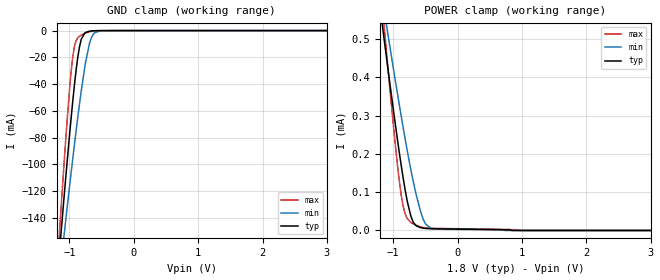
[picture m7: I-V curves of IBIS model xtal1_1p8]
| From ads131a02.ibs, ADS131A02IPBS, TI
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|   xtal1_1p8 Model
[Model]   xtal1_1p8
Model_type   Input
Vinl = 0.36
Vinh = 1.44
|   typ   min   max
|   (nom PVT)   (fast PVT)   (slow PVT)
C_comp   1.078e-12   1.074e-12   1.087e-12
| Where nom  PVT is Nominal Process, 1.8V, 27C
|   Fast PVT is Strong Process,  2V, -40C
|   Slow PVT is Weak Process,   1.65V, 125C
[Voltage Range]   1.8   1.65   2
|Junction Temperature
[Temperature Range]   27   125   -40
[Power Clamp Reference]   1.8   1.65   2
[GND Clamp Reference]   0   0   0
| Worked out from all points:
|   GND clamp passes 1 mA (typ) near -0.72 V on its own axis
[GND Clamp]
|   Voltage   I(typ)   I(min)   I(max)
-1.8V     -557.8mA   -477.6mA   -662.7mA
-1.148V   -161.8mA   -181.3mA   -146.5mA
-1.106V   -137.7mA   -162.9mA   -115.8mA
-1.055V   -108.9mA   -140.8mA   -79.9mA
-994mV    -76.12mA   -115mA     -41.72mA
-952.2mV  -54.96mA   -97.69mA   -21.36mA
-902mV    -32.17mA   -77.48mA   -8.397mA
-844.2mV  -12.42mA   -55.34mA   -4.36mA
-750.6mV  -1.441mA   -24.19mA   -1.867mA
-651.6mV  -231.6uA   -4.566mA   -469.7uA
-521.2mV  -19.95uA   -158.6uA   -32.31uA
3.6V      0A         0A         0A
[POWER Clamp]
|   Voltage   I(typ)   I(min)   I(max)
-1.8V     1.397mA    1.307mA    1.824mA
-1.371V   808.2uA    827.7uA    976.3uA
-1.141V   501uA      576.8uA    535.8uA
-1.098V   444.6uA    530.5uA    455.5uA
-975.6mV  289uA      401.3uA    238.9uA
-874mV    168.9uA    297.8uA    91.63uA
-812mV    104.5uA    237.5uA    42.77uA
-730mV    40.72uA    163.1uA    21.94uA
-644mV    12.78uA    94.68uA    13.6uA
-528mV    5.976uA    27.65uA    7.275uA
-404.1mV  4.46uA     5.019uA    5.573uA
3.6V      0A         0A         0A
